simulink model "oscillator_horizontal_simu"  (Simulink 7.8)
settings: Solver=ode45  StartTime=0.0  StopTime=10.0  RelTol=1e-3
undefined symbols (not defined in the file or in its folder): MP

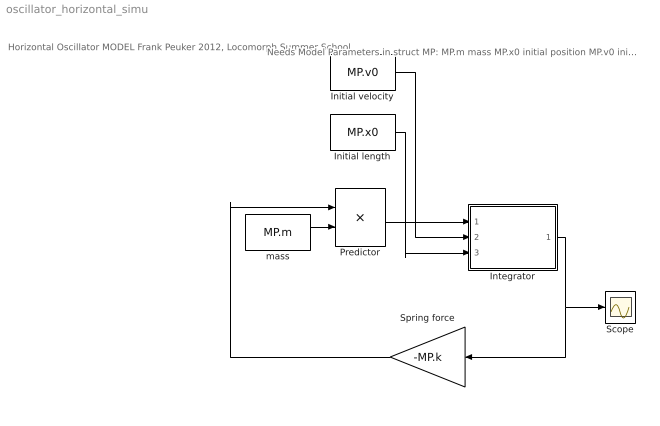
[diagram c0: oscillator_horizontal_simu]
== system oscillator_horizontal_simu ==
  note: Horizontal Oscillator MODEL Frank Peuker 2012, Locomorph Summer School
  note: Needs Model Parameters in struct MP: MP.m mass MP.x0 initial position MP.v0 initial speed MP.k stiffness of spring
  Initial length : Constant  Value=MP.x0
  Initial velocity : Constant  Value=MP.v0
  Integrator : Subsystem
  Predictor : Product  Inputs=*/
  Scope : Scope
  Spring force : Gain  Gain=-MP.k
  mass : Constant  Value=MP.m
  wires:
  Initial velocity/1 -> Integrator/2(v_init)
  Initial length/1 -> Integrator/3(L_init)
  Predictor/1 -> Integrator/1(a)
  mass/1 -> Predictor/2
  Integrator/1(L) -> Spring force/1, Scope/1
  Spring force/1 -> Predictor/1

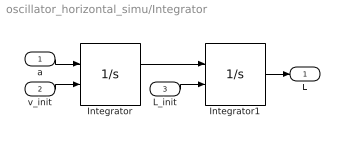
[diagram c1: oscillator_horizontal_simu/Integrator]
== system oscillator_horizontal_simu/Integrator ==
  a : Inport
  v_init : Inport  Port=2
  L_init : Inport  Port=3
  Integrator : Integrator  InitialConditionSource=external
  Integrator1 : Integrator  InitialConditionSource=external
  L : Outport
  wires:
  Integrator/1 -> Integrator1/1
  a/1 -> Integrator/1
  Integrator1/1 -> L/1
  v_init/1 -> Integrator/2
  L_init/1 -> Integrator1/2
